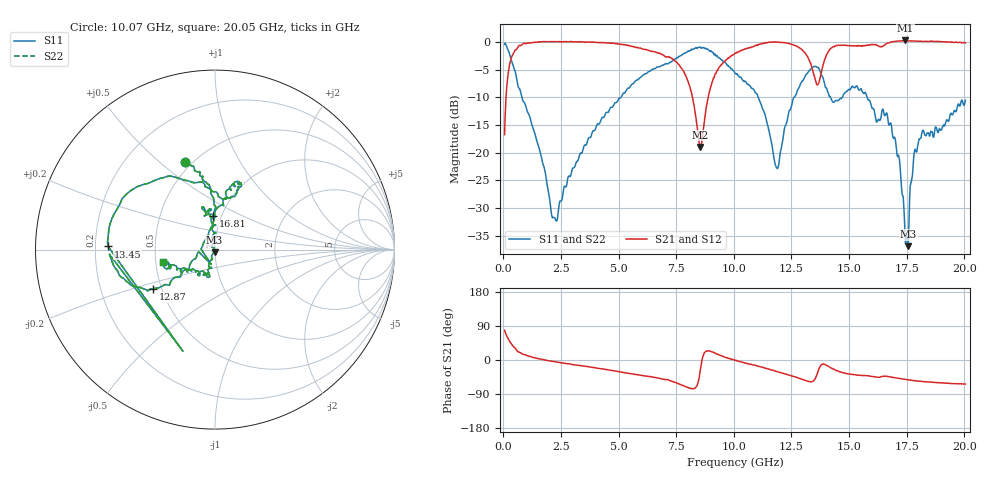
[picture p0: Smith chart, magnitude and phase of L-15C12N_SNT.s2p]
#	mhz	s	ma	r	50
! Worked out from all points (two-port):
!   1001 points, 50 MHz to 20.05 GHz, reference 50 ohm
!   highest |S21| = 0.27 dB at 17.45 GHz (marker M1); lowest = -18.9 dB at 8.55 GHz (marker M2)
!   |S21| within 3 dB of the highest: 354 MHz to 7.202 GHz (6.848 GHz wide, 181 % of centre); 13.99 GHz to end of sweep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
!   lowest |S11| = -36.9 dB at 17.57 GHz (marker M3), VSWR 1.03, Z = 49.8 - j1.41 ohm
!   |S11| at or under -10 dB: 804.9 MHz to 5.101 GHz (4.296 GHz wide, 145 % of centre); 11.05 GHz to 12.6 GHz (1.551 GHz wide, 13.1 % of centre); 15.79 GHz to end of sweep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
!   |S22| runs from -36.9 to -0.2 dB; largest |S21 - S12| = 0
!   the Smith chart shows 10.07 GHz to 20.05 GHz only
!   S11 on the Smith chart (normalised r, x): 10.07 GHz: 0.46, +0.61; 12.87 GHz: 0.45, -0.24; 13.45 GHz: 0.25, +0.01; 16.81 GHz: 0.92, +0.35; 20.05 GHz: 0.55, -0.09
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50  0.9537 171.6  0.1457 78.4  0.1457 78.4  0.9537 171.6
290  0.7436 140.7  0.6538 47.0  0.6538 47.0  0.7436 140.7
750  0.3501 116.4  0.9275 18.8  0.9275 18.8  0.3501 116.4
2190  0.02608 173.6  1.006 -4.3  1.006 -4.3  0.02608 173.6
3390  0.09863 -116.0  1.001 -15.2  1.001 -15.2  0.09863 -116.0
6730  0.5942 -136.9  0.7914 -48.0  0.7914 -48.0  0.5942 -136.9
7890  0.7949 -163.6  0.506 -69.8  0.506 -69.8  0.7949 -163.6
8550  0.8985 161.4  0.1131 -25.0  0.1131 -25.0  0.8985 161.4
10050  0.5247 110.2  0.7903 -0.6  0.7903 -0.6  0.5247 110.2
10070  0.5182 109.0  0.7894 -1.1  0.7894 -1.1  0.5182 109.0
11870  0.07245 157.7  0.9957 -30.7  0.9957 -30.7  0.07245 157.7
12870  0.4071 -147.6  0.8765 -49.0  0.8765 -49.0  0.4071 -147.6
13390  0.5836 -175.6  0.5877 -57.2  0.5877 -57.2  0.5836 -175.6
13450  0.5959 178.3  0.5278 -55.5  0.5278 -55.5  0.5959 178.3
13850  0.4842 122.2  0.5937 -11.1  0.5937 -11.1  0.4842 122.2
14430  0.2972 76.9  0.9243 -27.4  0.9243 -27.4  0.2972 76.9
16730  0.1779 94.7  0.9816 -44.1  0.9816 -44.1  0.1779 94.7
16810  0.1854 93.1  0.9933 -44.8  0.9933 -44.8  0.1854 93.1
17450  0.01523 -149.3  1.032 -51.2  1.032 -51.2  0.01523 -149.3
17570  0.01436 -98.3  1.02 -52.3  1.02 -52.3  0.01436 -98.3
18130  0.1387 -108.5  1.012 -56.4  1.012 -56.4  0.1387 -108.5
20050  0.298 -166.1  0.9823 -63.5  0.9823 -63.5  0.298 -166.1
